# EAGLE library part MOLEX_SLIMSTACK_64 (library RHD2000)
Molex 64-pin SlimStack connector (DigiKey WM24076-ND)
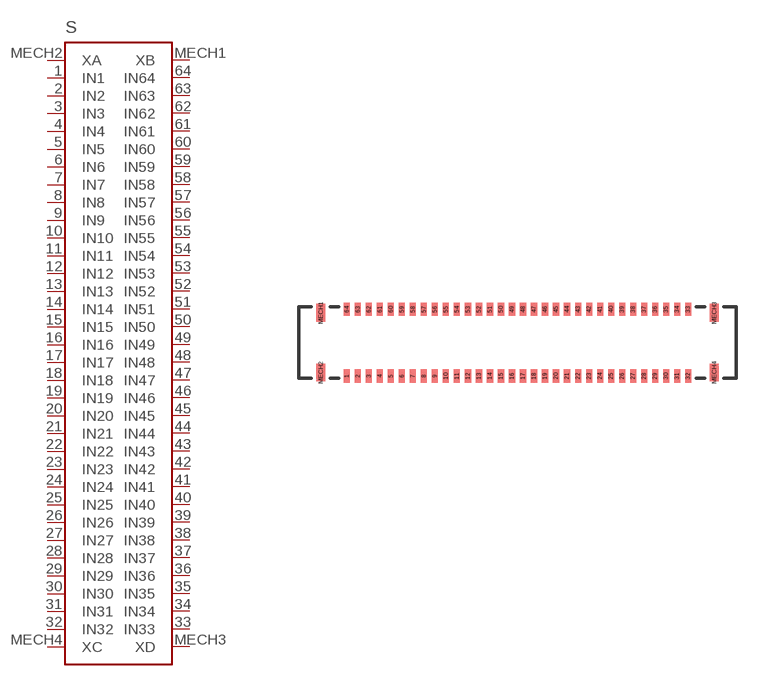
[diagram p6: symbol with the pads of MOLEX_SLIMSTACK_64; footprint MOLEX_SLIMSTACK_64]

Designator prefix S

## MOLEX_SLIMSTACK_64  [MOLEX_SLIMSTACK_64]
1  IN1  in
2  IN2  in
3  IN3  in
4  IN4  in
5  IN5  in
6  IN6  in
7  IN7  in
8  IN8  in
9  IN9  in
10  IN10  in
11  IN11  in
12  IN12  in
13  IN13  in
14  IN14  in
15  IN15  in
16  IN16  in
17  IN17  in
18  IN18  in
19  IN19  in
20  IN20  in
21  IN21  in
22  IN22  in
23  IN23  in
24  IN24  in
25  IN25  in
26  IN26  in
27  IN27  in
28  IN28  in
29  IN29  in
30  IN30  in
31  IN31  in
32  IN32  in
33  IN33  in
34  IN34  in
35  IN35  in
36  IN36  in
37  IN37  in
38  IN38  in
39  IN39  in
40  IN40  in
41  IN41  in
42  IN42  in
43  IN43  in
44  IN44  in
45  IN45  in
46  IN46  in
47  IN47  in
48  IN48  in
49  IN49  in
50  IN50  in
51  IN51  in
52  IN52  in
53  IN53  in
54  IN54  in
55  IN55  in
56  IN56  in
57  IN57  in
58  IN58  in
59  IN59  in
60  IN60  in
61  IN61  in
62  IN62  in
63  IN63  in
64  IN64  in
MECH1  XB  in
MECH2  XA  in
MECH3  XD  in
MECH4  XC  in

## Footprint MOLEX_SLIMSTACK_64 (pad centres in mm)
Molex SlimStack 64-pin connector (DigiKey part WM24076-ND)
smd 0.22 x 0.475: 1 -6.2,-1.212; 2 -5.8,-1.212; 3 -5.4,-1.212; 4 -5,-1.212; 5 -4.6,-1.212; 6 -4.2,-1.212; 7 -3.8,-1.212; 8 -3.4,-1.212; 9 -3,-1.212; 10 -2.6,-1.212; 11 -2.2,-1.212; 12 -1.8,-1.212; 13 -1.4,-1.212; 14 -1,-1.212; 15 -0.6,-1.212; 16 -0.2,-1.212; 17 0.2,-1.212; 18 0.6,-1.212; 19 1,-1.212; 20 1.4,-1.212; 21 1.8,-1.212; 22 2.2,-1.212; 23 2.6,-1.212; 24 3,-1.212; 25 3.4,-1.212; 26 3.8,-1.212; 27 4.2,-1.212; 28 4.6,-1.212; 29 5,-1.212; 30 5.4,-1.212; 31 5.8,-1.212; 32 6.2,-1.212; 33 6.2,1.212; 34 5.8,1.212; 35 5.4,1.212; 36 5,1.212; 37 4.6,1.212; 38 4.2,1.212; 39 3.8,1.212; 40 3.4,1.212; 41 3,1.212; 42 2.6,1.212; 43 2.2,1.212; 44 1.8,1.212; 45 1.4,1.212; 46 1,1.212; 47 0.6,1.212; 48 0.2,1.212; 49 -0.2,1.212; 50 -0.6,1.212; 51 -1,1.212; 52 -1.4,1.212; 53 -1.8,1.212; 54 -2.2,1.212; 55 -2.6,1.212; 56 -3,1.212; 57 -3.4,1.212; 58 -3.8,1.212; 59 -4.2,1.212; 60 -4.6,1.212; 61 -5,1.212; 62 -5.4,1.212; 63 -5.8,1.212; 64 -6.2,1.212
smd 0.32 x 0.65: MECH1 -7.15,1.085; MECH2 -7.15,-1.085; MECH3 7.15,1.085; MECH4 7.15,-1.085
